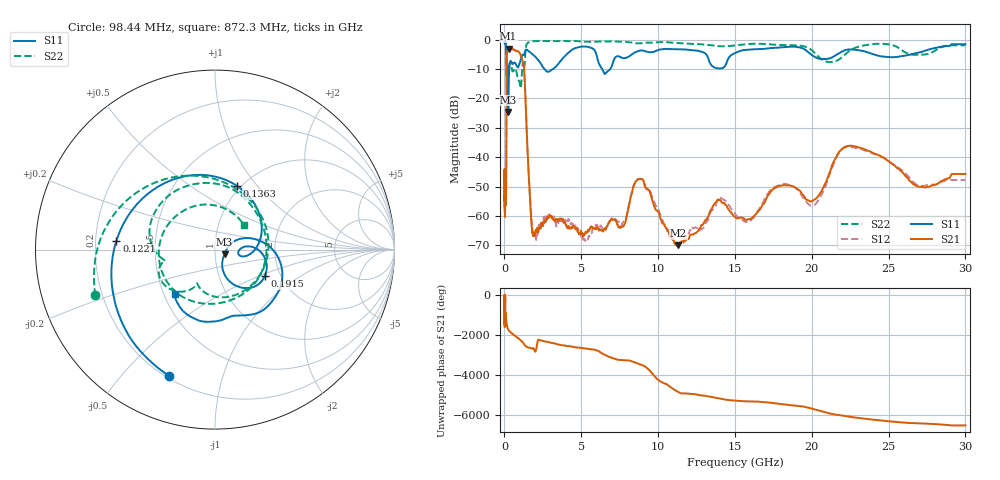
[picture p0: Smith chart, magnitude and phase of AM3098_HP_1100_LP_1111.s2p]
! Date/Time: Thu, Feb 28, 2019 8:45 AM
! Network Analyzer: Agilent Technologies E8364B Rev: A.07.50.67
! Sweep from 0.010 to 30.000 GHz, 1601 Points, Sweep Type: LOG
! Power Supply: 5.023 V, 0.002 A
# Hz S DB R 50
!freq MagS11 AngS11 MagS21 AngS21 MagS12 AngS12 MagS22 AngS22
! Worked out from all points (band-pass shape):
!   1601 points, 10 MHz to 30 GHz, reference 50 ohm
!   highest |S21| = -3.12 dB at 263.8 MHz (marker M1); lowest = -70.0 dB at 11.31 GHz (marker M2)
!   |S21| within 3 dB of the highest: 149.2 MHz to 1.112 GHz (963.2 MHz wide, 153 % of centre)
!   lowest |S11| = -24.6 dB at 247.2 MHz (marker M3), VSWR 1.12, Z = 55.5 - j2.84 ohm
!   |S11| at or under -10 dB: 140.1 MHz to 309.3 MHz (169.1 MHz wide, 75.3 % of centre); 2.601 GHz to 3.173 GHz (571.7 MHz wide, 19.8 % of centre); 6.355 GHz to 6.894 GHz (539.1 MHz wide, 8.14 % of centre)
!   |S22| runs from -16.5 to -0.5 dB; largest |S21 - S12| = 0.012
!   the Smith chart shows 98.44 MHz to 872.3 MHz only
!   S11 on the Smith chart (normalised r, x): 98.44 MHz: 0.21, -0.68; 122.1 MHz: 0.29, +0.04; 136.3 MHz: 0.96, +0.79; 191.5 MHz: 1.66, -0.54; 872.3 MHz: 0.57, -0.32
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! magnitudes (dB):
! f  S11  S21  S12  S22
! 10 MHz  -0.3  -45.0  -44.3  -0.6
! 38.04 MHz  -0.4  -60.0  -56.8  -0.9
! 98.44 MHz  -2.5  -52.9  -53.3  -2.9
! 122.1 MHz  -5.2  -34.1  -34.2  -6.7
! 136.3 MHz  -8.5  -13.3  -13.2  -10.8
! 144.7 MHz  -12.3  -7.5  -7.4  -11.8
! 191.5 MHz  -10.1  -3.8  -3.8  -9.3
! 247.2 MHz  -24.6  -3.2  -3.1  -10.9
! 263.8 MHz  -19.1  -3.1  -3.1  -10.7
! 332.1 MHz  -8.5  -3.4  -3.3  -8.3
! 550.5 MHz  -8.2  -3.4  -3.3  -10.8
! 872.3 MHz  -9.5  -4.0  -4.0  -13.5
! 1.27 GHz  -5.3  -9.7  -9.7  -9.9
! 1.758 GHz  -4.7  -62.1  -61.0  -0.7
! 2.084 GHz  -6.3  -65.5  -66.9  -0.5
! 7.926 GHz  -6.2  -60.9  -60.4  -0.8
! 8.893 GHz  -3.7  -47.4  -47.4  -1.3
! 11.31 GHz  -3.3  -70.0  -69.8  -1.2
! 14.02 GHz  -9.9  -54.5  -54.2  -2.3
! 20.1 GHz  -5.6  -54.7  -56.4  -4.1
! 22.56 GHz  -3.4  -36.1  -36.6  -3.5
! 30 GHz  -1.6  -45.7  -47.8  -2.0
